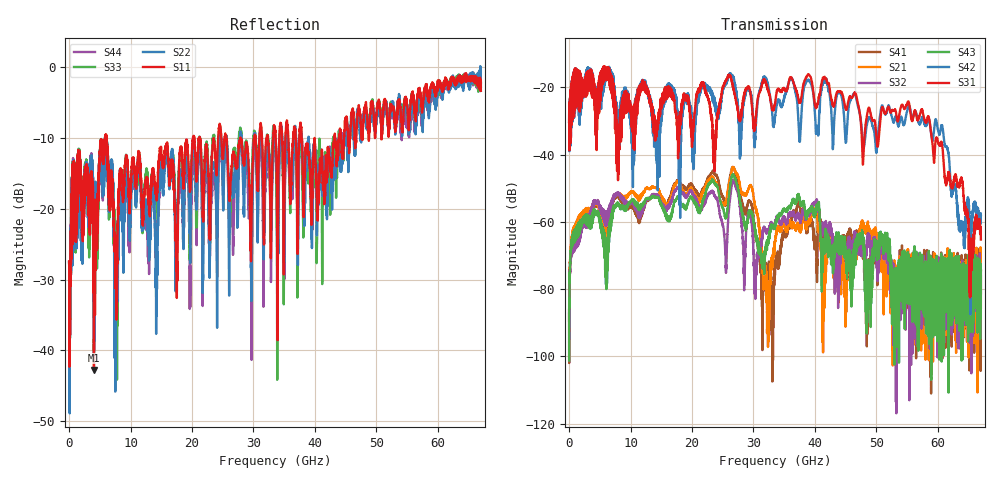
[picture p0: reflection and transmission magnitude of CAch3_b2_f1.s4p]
!Agilent Technologies,N5247A,US51170199,A.09.90.13
!Agilent N5247A: A.09.90.13
!Date: Thursday, October 18, 2018 12:01:04
!Correction: S11(Full 4 Port(1,2,3,4))
!S12(Full 4 Port(1,2,3,4))
!S13(Full 4 Port(1,2,3,4))
!S14(Full 4 Port(1,2,3,4))
!S21(Full 4 Port(1,2,3,4))
!S22(Full 4 Port(1,2,3,4))
!S23(Full 4 Port(1,2,3,4))
!S24(Full 4 Port(1,2,3,4))
!S31(Full 4 Port(1,2,3,4))
!S32(Full 4 Port(1,2,3,4))
!S33(Full 4 Port(1,2,3,4))
!S34(Full 4 Port(1,2,3,4))
!S41(Full 4 Port(1,2,3,4))
!S42(Full 4 Port(1,2,3,4))
!S43(Full 4 Port(1,2,3,4))
!S44(Full 4 Port(1,2,3,4))
!S4P File: Measurements: <S11,S12,S13,S14>,
!<S21,S22,S23,S24>,
!<S31,S32,S33,S34>,
!<S41,S42,S43,S44>:
# Hz S  dB  R 50
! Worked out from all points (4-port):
!   6701 points, 10 MHz to 67 GHz, reference 50 ohm
!   strongest paths, dB at 10 MHz, 16.76 GHz, 33.51 GHz, 50.25 GHz, 67 GHz:
!     S31: -30.2, -22.3, -24.8, -37.3, -65.3
!     S42: -30.3, -20.1, -28.5, -34.3, -58.2
!     S43: -101.2, -57.0, -60.7, -67.4, -74.4
!     S32: -87.1, -53.3, -60.4, -70.1, -76.2
!     S21: -87.6, -51.9, -65.8, -67.2, -85.4
!     S41: -86.1, -50.7, -72.8, -75.0, -74.6
!   lowest |S11| = -42.7 dB at 4.049 GHz (marker M1), VSWR 1.01, Z = 49.4 - j0.444 ohm
!   |S11| at or under -10 dB: start of sweep to 5.856 GHz; 6.122 GHz to 20.16 GHz (14.04 GHz wide, 107 % of centre); 39.93 GHz to 43.16 GHz (3.234 GHz wide, 7.79 % of centre)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
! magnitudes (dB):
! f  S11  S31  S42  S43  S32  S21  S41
! 10 MHz  -27.4  -30.2  -30.3  -101.2  -87.1  -87.6  -86.1
! 4.049 GHz  -42.7  -21.4  -20.4  -56.3  -53.6  -53.8  -54.0
! 26.72 GHz  -12.0  -20.2  -16.8  -45.8  -47.6  -43.7  -43.8
! 32.42 GHz  -10.8  -21.0  -19.7  -65.2  -62.4  -84.5  -77.3
! 37.3 GHz  -15.5  -23.4  -29.2  -52.0  -58.0  -61.3  -54.0
! 55.11 GHz  -6.6  -24.3  -26.4  -72.1  -72.8  -72.4  -72.9
! 67 GHz  -3.3  -65.3  -58.2  -74.4  -76.2  -85.4  -74.6
